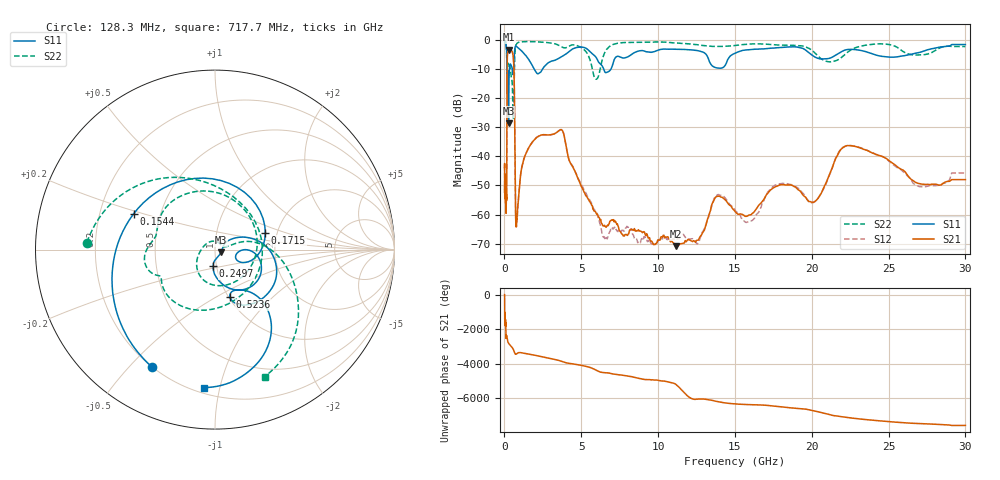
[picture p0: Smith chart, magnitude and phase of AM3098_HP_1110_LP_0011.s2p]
! Date/Time: Thu, Feb 28, 2019 8:46 AM
! Network Analyzer: Agilent Technologies E8364B Rev: A.07.50.67
! Sweep from 0.010 to 30.000 GHz, 1601 Points, Sweep Type: LOG
! Power Supply: 5.022 V, 0.002 A
# Hz S DB R 50
!freq MagS11 AngS11 MagS21 AngS21 MagS12 AngS12 MagS22 AngS22
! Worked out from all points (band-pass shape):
!   1601 points, 10 MHz to 30 GHz, reference 50 ohm
!   highest |S21| = -3.40 dB at 277.3 MHz (marker M1); lowest = -70.8 dB at 11.14 GHz (marker M2)
!   |S21| within 3 dB of the highest: 183.4 MHz to 581.7 MHz (398.3 MHz wide, 104 % of centre)
!   lowest |S11| = -28.7 dB at 263.8 MHz (marker M3), VSWR 1.08, Z = 53.4 - j1.64 ohm
!   |S11| at or under -10 dB: 170 MHz to 321.3 MHz (151.3 MHz wide, 61.6 % of centre); 1.92 GHz to 2.495 GHz (574.8 MHz wide, 26 % of centre); 6.455 GHz to 6.941 GHz (485.8 MHz wide, 7.25 % of centre)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
!   |S22| runs from -27.4 to -0.5 dB; largest |S21 - S12| = 0.012
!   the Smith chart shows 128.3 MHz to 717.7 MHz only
!   S11 on the Smith chart (normalised r, x): 128.3 MHz: 0.20, -0.58; 154.4 MHz: 0.35, +0.18; 171.5 MHz: 1.73, +0.35; 249.7 MHz: 0.96, -0.18; 523.6 MHz: 1.01, -0.58; 717.7 MHz: 0.24, -0.90
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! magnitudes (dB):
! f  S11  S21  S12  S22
! 10 MHz  -0.3  -43.9  -42.9  -0.5
! 38.04 MHz  -0.3  -50.3  -51.4  -0.7
! 128.3 MHz  -2.6  -53.0  -54.5  -2.9
! 144.7 MHz  -4.3  -51.9  -51.2  -5.7
! 154.4 MHz  -6.1  -36.1  -35.9  -10.2
! 171.5 MHz  -10.6  -11.5  -11.5  -8.8
! 249.7 MHz  -20.8  -3.6  -3.5  -9.0
! 263.8 MHz  -28.7  -3.5  -3.4  -9.3
! 277.3 MHz  -20.7  -3.4  -3.4  -9.4
! 335.4 MHz  -9.1  -3.5  -3.5  -8.9
! 523.6 MHz  -11.2  -4.5  -4.5  -17.6
! 550.5 MHz  -12.0  -5.1  -5.1  -25.1
! 633.3 MHz  -6.0  -13.7  -13.6  -12.6
! 717.7 MHz  -2.3  -56.8  -57.4  -2.4
! 2.084 GHz  -11.4  -33.6  -33.5  -0.7
! 3.742 GHz  -5.8  -31.0  -31.0  -2.5
! 6.488 GHz  -10.5  -63.7  -67.6  -4.9
! 7.926 GHz  -6.1  -66.8  -64.5  -1.0
! 11.14 GHz  -3.3  -70.8  -68.4  -1.1
! 20.1 GHz  -5.6  -55.8  -55.8  -4.1
! 22.56 GHz  -3.3  -36.4  -36.3  -3.5
! 30 GHz  -1.7  -48.0  -45.7  -2.4
